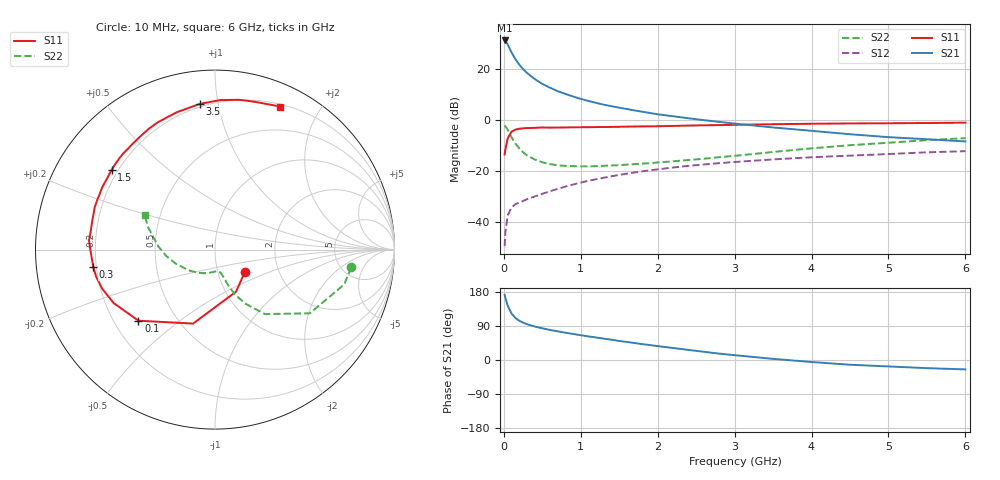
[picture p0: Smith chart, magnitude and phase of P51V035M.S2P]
! SIEMENS Small Signal Semiconductors
! BFP183
! Si NPN RF Bipolar Junction Transistor in SOT143
! VCE = 1 V  IC = 35 mA
! Common Emitter S-Parameters:  March  1996
# GHz  S  MA  R  50
!  f  S11  S21  S12  S22
! GHz  MAG  ANG  MAG  ANG  MAG  ANG  MAG  ANG
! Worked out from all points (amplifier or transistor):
!   36 points, 10 MHz to 6 GHz, reference 50 ohm
!   highest |S21| = 31.1 dB at 10 MHz (marker M1)
!   |S21| within 3 dB of that: start of sweep to 72.58 MHz
!   unconditionally stable (mu >= 1): start of sweep to 18.22 MHz; 251.7 MHz to end of sweep
!   at 250 MHz: K = 1.00, MSG = 25.9 dB, |S12| = -31.9 dB
!   at 1.4 GHz: K = 1.67, MAG = 9.0 dB, |S12| = -22.2 dB
!   at 6 GHz: K = 1.31, MAG = -1.4 dB, |S12| = -12.3 dB
!   S11 on the Smith chart (normalised r, x): 10 MHz: 1.35, -0.35; 100 MHz: 0.30, -0.36; 300 MHz: 0.19, -0.07; 1.5 GHz: 0.18, +0.33; 3.5 GHz: 0.18, +0.89; 6 GHz: 0.22, +1.53
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0.01  0.2077 -36.6  35.96 171.9  0.0033 76.7  0.7656 -7.4
0.02  0.2621 -63.4  35.15 164.1  0.0062 73.1  0.7456 -15.1
0.05  0.4299 -106.5  29.93 143.5  0.0132 60.2  0.6364 -33.9
0.1  0.5819 -137.1  20.91 122.6  0.019 45.8  0.4539 -52.3
0.15  0.6385 -152.2  15.5 111.0  0.0219 43.1  0.342 -61.0
0.2  0.6654 -161.0  12.1 103.7  0.0237 42.1  0.2743 -65.8
0.25  0.6791 -167.2  9.845 98.5  0.0254 43.3  0.2303 -68.6
0.3  0.6852 -172.0  8.324 94.6  0.0274 45.0  0.2004 -70.3
0.4  0.6927 -179.0  6.316 88.4  0.0311 48.2  0.1661 -72.4
0.5  0.7038 175.8  5.044 83.6  0.0352 51.0  0.1463 -74.3
0.6  0.6999 171.7  4.246 79.3  0.0395 53.1  0.1347 -76.2
0.7  0.7021 167.2  3.635 75.6  0.044 54.7  0.1275 -78.3
0.8  0.7048 164.0  3.209 72.0  0.0487 55.4  0.1242 -80.1
1  0.7121 157.0  2.564 65.4  0.0583 56.5  0.1216 -85.0
1.1  0.7134 153.9  2.335 62.2  0.0635 56.7  0.1217 -87.8
1.5  0.7273 142.4  1.721 50.2  0.0827 55.0  0.1283 -99.1
2.2  0.7552 123.7  1.17 31.6  0.1154 49.0  0.1527 -121.6
2.8  0.7845 109.6  0.907 16.8  0.1406 42.5  0.1842 -140.9
3.5  0.8163 95.9  0.705 3.0  0.1664 35.4  0.2329 -160.5
4.5  0.8456 80.8  0.519 -12.5  0.1975 24.8  0.3164 176.8
5.5  0.8618 70.0  0.414 -21.5  0.2293 15.6  0.3969 161.0
6  0.8759 65.5  0.375 -24.8  0.2413 10.4  0.4355 153.9
